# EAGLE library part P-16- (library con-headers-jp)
HEADER PLUG PINS
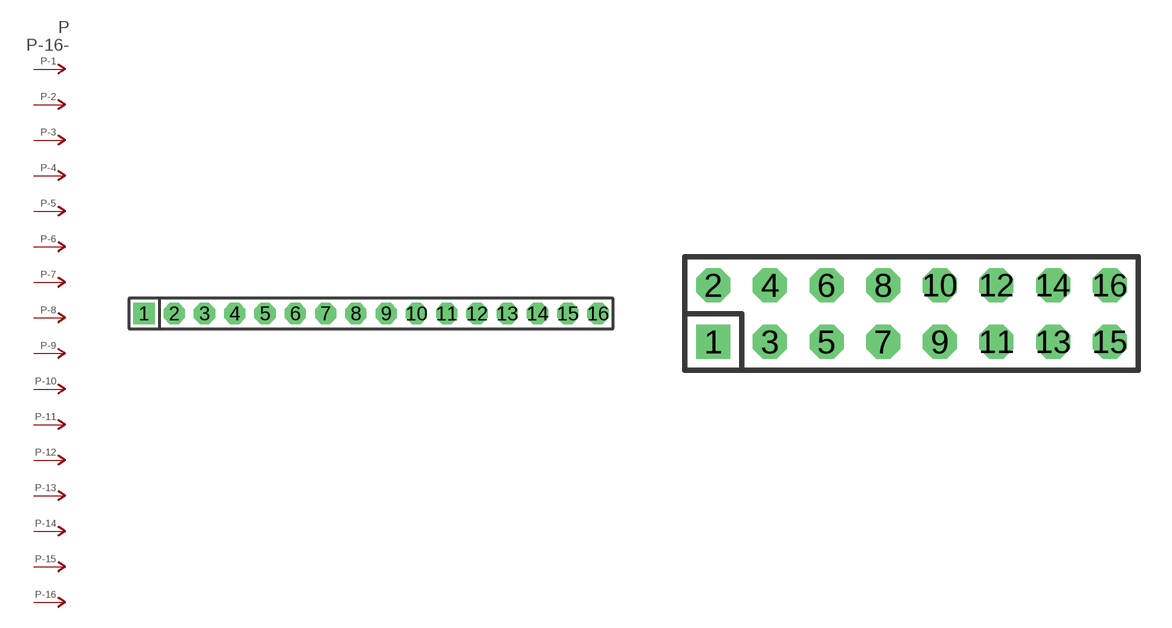
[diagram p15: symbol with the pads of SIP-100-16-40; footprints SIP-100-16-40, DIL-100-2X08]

Designator prefix P; gates -2=P-N -3=P-N -4=P-N -5=P-N -6=P-N -7=P-N -8=P-N -9=P-N -10=P-N -11=P-N -12=P-N -13=P-N -14=P-N -15=P-N -16=P-N -1=P-NV

## P-16-SIP-100-40  [SIP-100-16-40]
1  -1:P  pas
2  -2:P  pas
3  -3:P  pas
4  -4:P  pas
5  -5:P  pas
6  -6:P  pas
7  -7:P  pas
8  -8:P  pas
9  -9:P  pas
10  -10:P  pas
11  -11:P  pas
12  -12:P  pas
13  -13:P  pas
14  -14:P  pas
15  -15:P  pas
16  -16:P  pas

## P-16-100-2X08  [DIL-100-2X08]
Pads as for SIP-100-16-40

## P-16-100-2X08_M  [DIL-100-2X08_M]
Pads as for SIP-100-16-40

## P-16-2MM-2X08  [DIL-2MM-2X08]
Pads as for SIP-100-16-40

## P-16-2MM-2X08_M  [DIL-2MM-2X08_M]
Pads as for SIP-100-16-40

## P-16-SIP-100-32  [SIP-100-16-32]
Pads as for SIP-100-16-40

## P-16-SIP-100-40Y  [SIP-100-16-40Y]
Pads as for SIP-100-16-40

## P-16-SIP-100-32Y  [SIP-100-16-32Y]
Pads as for SIP-100-16-40

## P-16-LCW-116-XX-X-S  [LCW-116-XX-X-S]
Pads as for SIP-100-16-40

## P-16-LCW-116-XX-X-S-RE  [LCW-116-XX-X-S-RE]
Pads as for SIP-100-16-40

## Footprint SIP-100-16-40 (pad centres in mm)
SIP Header - 0.1", 40 mil drill
drill 1.016 pad 1.778 square: 1 -19.05,0
drill 1.016 pad 1.778 octagon: 2 -16.51,0; 3 -13.97,0; 4 -11.43,0; 5 -8.89,0; 6 -6.35,0; 7 -3.81,0; 8 -1.27,0; 9 1.27,0; 10 3.81,0; 11 6.35,0; 12 8.89,0; 13 11.43,0; 14 13.97,0; 15 16.51,0; 16 19.05,0

## Footprint DIL-100-2X08 (pad centres in mm)
PIN HEADER - 0.1"
drill 1.016 square: 1 -8.89,-1.27
drill 1.016 octagon: 2 -8.89,1.27; 3 -6.35,-1.27; 4 -6.35,1.27; 5 -3.81,-1.27; 6 -3.81,1.27; 7 -1.27,-1.27; 8 -1.27,1.27; 9 1.27,-1.27; 10 1.27,1.27; 11 3.81,-1.27; 12 3.81,1.27; 13 6.35,-1.27; 14 6.35,1.27; 15 8.89,-1.27; 16 8.89,1.27

## Footprint DIL-100-2X08_M (pad centres in mm)
PIN HEADER - MIRRORED 0.1"
drill 1.016 square: 1 -8.89,1.27
drill 1.016 octagon: 2 -8.89,-1.27; 3 -6.35,1.27; 4 -6.35,-1.27; 5 -3.81,1.27; 6 -3.81,-1.27; 7 -1.27,1.27; 8 -1.27,-1.27; 9 1.27,1.27; 10 1.27,-1.27; 11 3.81,1.27; 12 3.81,-1.27; 13 6.35,1.27; 14 6.35,-1.27; 15 8.89,1.27; 16 8.89,-1.27

## Footprint DIL-2MM-2X08 (pad centres in mm)
PIN HEADER - 2MM"
drill 0.711 square: 1 -7,-1
drill 0.711: 2 -7,1; 3 -5,-1; 4 -5,1; 5 -3,-1; 6 -3,1; 7 -1,-1; 8 -1,1; 9 1,-1; 10 1,1; 11 3,-1; 12 3,1; 13 5,-1; 14 5,1; 15 7,-1; 16 7,1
